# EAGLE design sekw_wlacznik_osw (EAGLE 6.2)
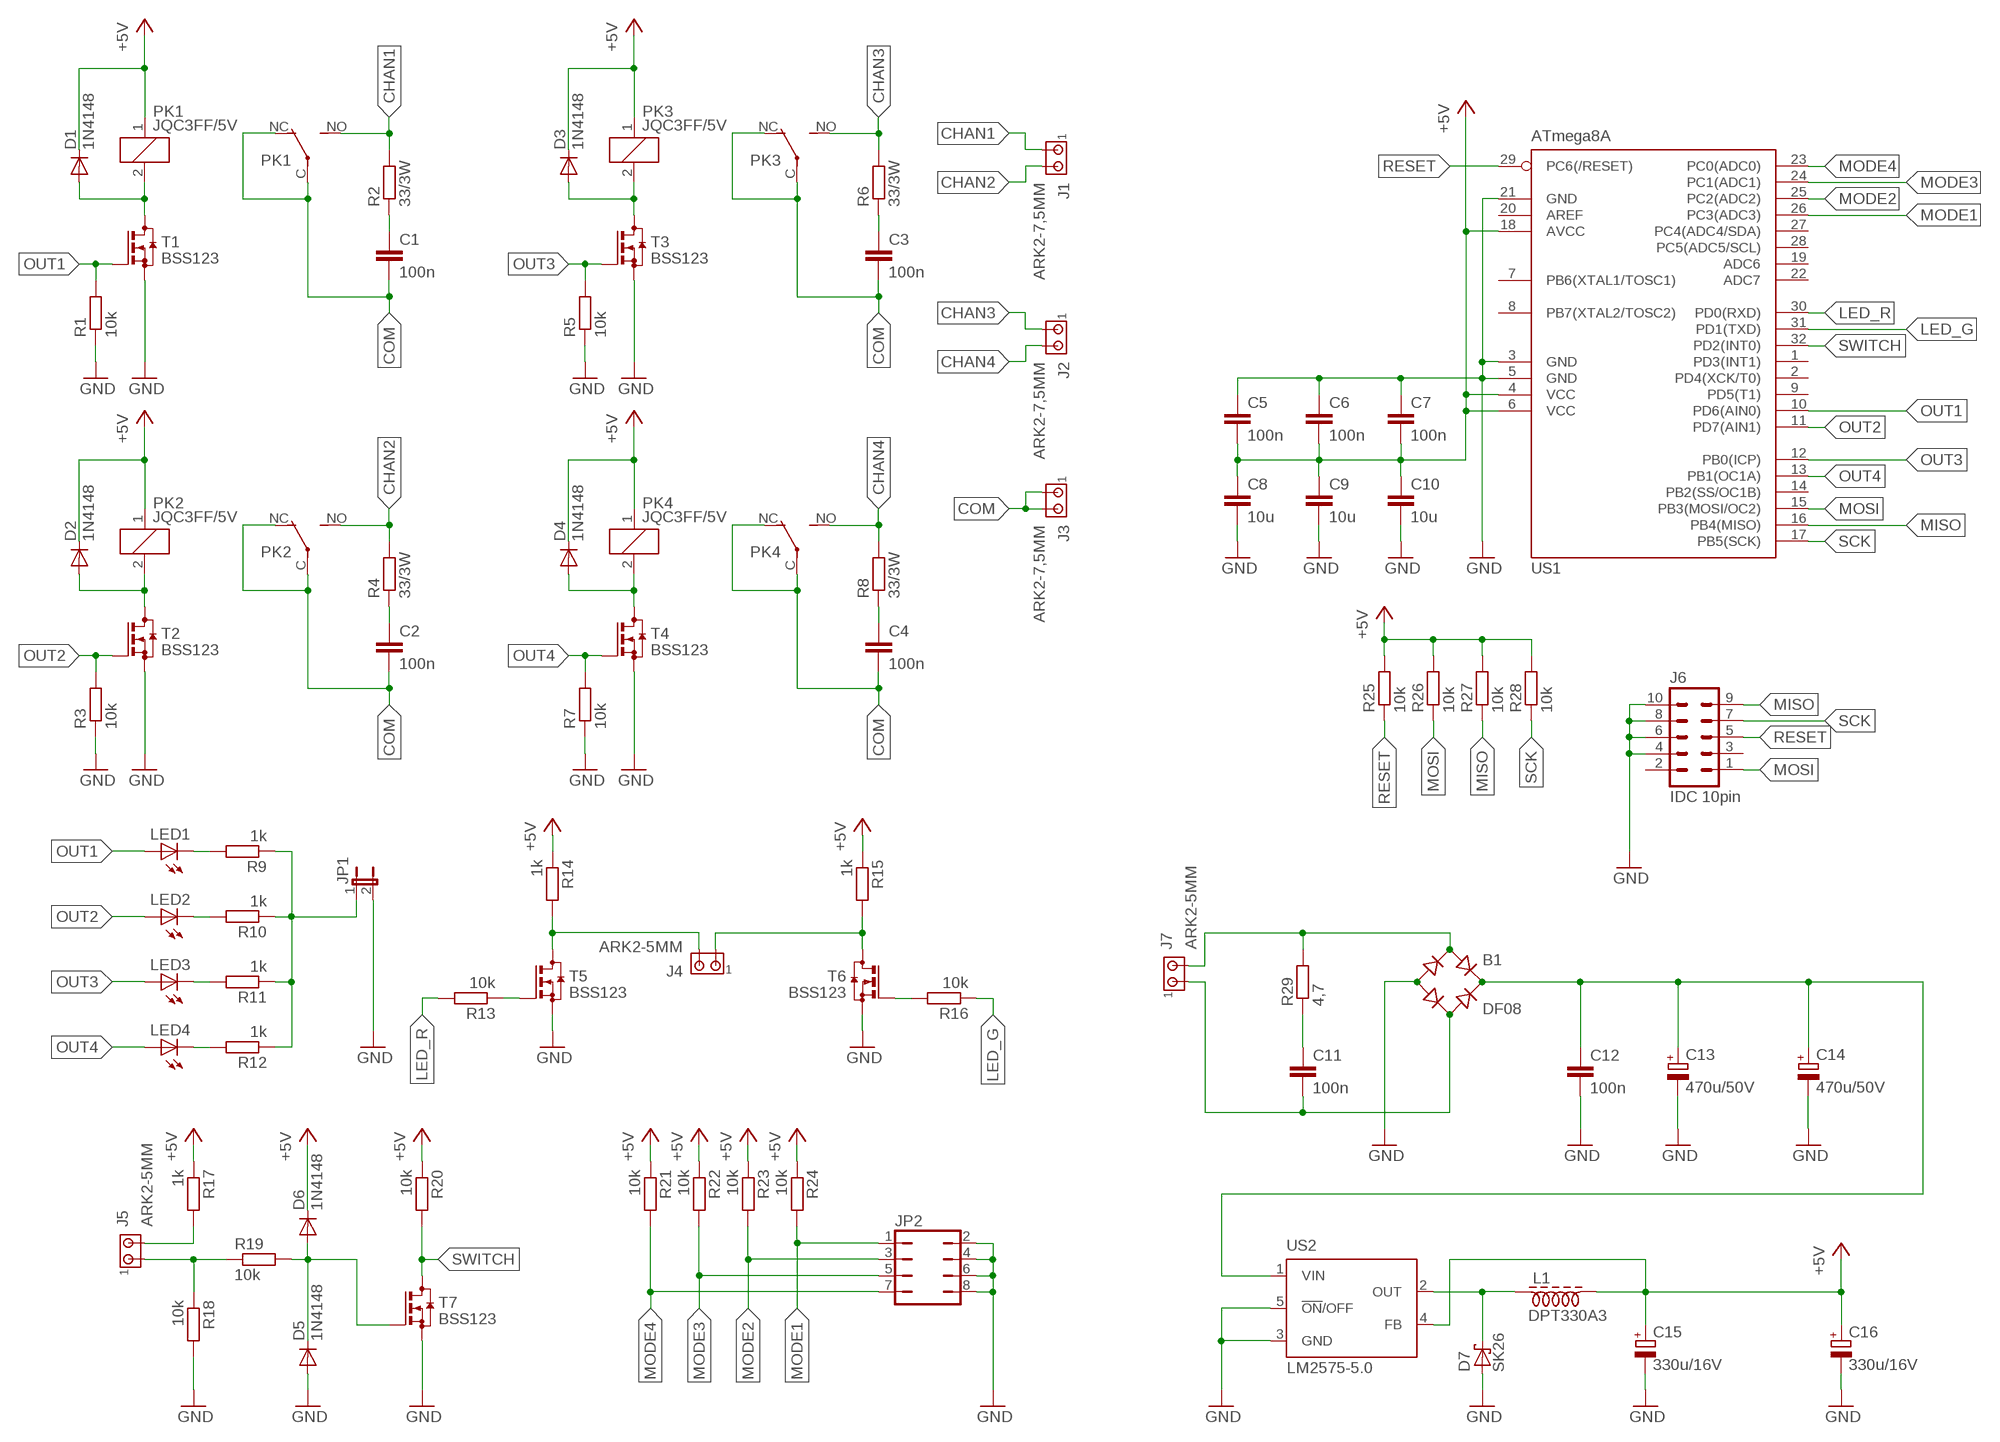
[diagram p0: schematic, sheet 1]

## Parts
B1  DF08  B-DIL  [B-DIL]
C1  100n  C-EU102_152-062X184  [C102_152-062X184]
C2  100n  C-EU102_152-062X184  [C102_152-062X184]
C3  100n  C-EU102_152-062X184  [C102_152-062X184]
C4  100n  C-EU102_152-062X184  [C102_152-062X184]
C5  100n  C-EUC0805  [C0805]
C6  100n  C-EUC0805  [C0805]
C7  100n  C-EUC0805  [C0805]
C8  10u  C-EUC0805  [C0805]
C9  10u  C-EUC0805  [C0805]
C10  10u  C-EUC0805  [C0805]
C11  100n  C-EUC0805  [C0805]
C12  100n  C-EUC0805  [C0805]
C13  470u/50V  CPOL-EUE5-10.5  [E5-10,5]
C14  470u/50V  CPOL-EUE5-10.5  [E5-10,5]
C15  330u/16V  CPOL-EUE3.5-8  [E3,5-8]
C16  330u/16V  CPOL-EUE3.5-8  [E3,5-8]
D1  1N4148  DIODE-MINIMELF  [MINIMELF]
D2  1N4148  DIODE-MINIMELF  [MINIMELF]
D3  1N4148  DIODE-MINIMELF  [MINIMELF]
D4  1N4148  DIODE-MINIMELF  [MINIMELF]
D5  1N4148  DIODE-MINIMELF  [MINIMELF]
D6  1N4148  DIODE-MINIMELF  [MINIMELF]
D7  SK26  SCHOTTKY-DIODESMD  [SMB]
J1  ARK2-7,5MM  [2PIN-7,5MM]
J2  ARK2-7,5MM  [2PIN-7,5MM]
J3  ARK2-7,5MM  [2PIN-7,5MM]
J4  ARK2-5MM  [2PIN-5MM]
J5  ARK2-5MM  [2PIN-5MM]
J6  IDC 10pin  ML10  [ML10]
J7  ARK2-5MM  [2PIN-5MM]
JP1  JP1E  [JP1]
JP2  JP4Q  [JP4Q]
L1  DPT330A3  DLAWIK-TOROID_16,5X9MM  [L_TOROID_16,5X9MM]
LED1  LEDCHIPLED_0805  [CHIPLED_0805]
LED2  LEDCHIPLED_0805  [CHIPLED_0805]
LED3  LEDCHIPLED_0805  [CHIPLED_0805]
LED4  LEDCHIPLED_0805  [CHIPLED_0805]
PK1  JQC3FF/5V  PK_POJED-JQC-3FG  [PK_POJED_JQC-3FG]
PK2  JQC3FF/5V  PK_POJED-JQC-3FG  [PK_POJED_JQC-3FG]
PK3  JQC3FF/5V  PK_POJED-JQC-3FG  [PK_POJED_JQC-3FG]
PK4  JQC3FF/5V  PK_POJED-JQC-3FG  [PK_POJED_JQC-3FG]
R1  10k  R-EU_R0805  [R0805]
R2  33/3W  R-EU_0613/5V  [P0613V]
R3  10k  R-EU_R0805  [R0805]
R4  33/3W  R-EU_0613/5V  [P0613V]
R5  10k  R-EU_R0805  [R0805]
R6  33/3W  R-EU_0613/5V  [P0613V]
R7  10k  R-EU_R0805  [R0805]
R8  33/3W  R-EU_0613/5V  [P0613V]
R9  1k  R-EU_R0805  [R0805]
R10  1k  R-EU_R0805  [R0805]
R11  1k  R-EU_R0805  [R0805]
R12  1k  R-EU_R0805  [R0805]
R13  10k  R-EU_R0805  [R0805]
R14  1k  R-EU_R0805  [R0805]
R15  1k  R-EU_R0805  [R0805]
R16  10k  R-EU_R0805  [R0805]
R17  1k  R-EU_R0805  [R0805]
R18  10k  R-EU_R0805  [R0805]
R19  10k  R-EU_R0805  [R0805]
R20  10k  R-EU_R0805  [R0805]
R21  10k  R-EU_R0805  [R0805]
R22  10k  R-EU_R0805  [R0805]
R23  10k  R-EU_R0805  [R0805]
R24  10k  R-EU_R0805  [R0805]
R25  10k  R-EU_R0805  [R0805]
R26  10k  R-EU_R0805  [R0805]
R27  10k  R-EU_R0805  [R0805]
R28  10k  R-EU_R0805  [R0805]
R29  4,7  R-EU_M1206  [M1206]
T1  BSS123  [SOT23]
T2  BSS123  [SOT23]
T3  BSS123  [SOT23]
T4  BSS123  [SOT23]
T5  BSS123  [SOT23]
T6  BSS123  [SOT23]
T7  BSS123  [SOT23]
US1  ATmega8A  MEGA8-AI  [TQFP32-08]
US2  LM2575-5.0  LM2596T  [T05D]

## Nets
+5V: C5.2 C6.2 C7.2 C8.1 C9.1 C10.1 C15.+ C16.+ D1.C D2.C D3.C D4.C D6.C L1.P$2 PK1.1 PK2.1 PK3.1 PK4.1 R14.1 R15.1 R17.1 R20.1 R21.1 R22.1 R23.1 R24.1 R25.2 R26.2 R27.2 R28.2 US1.4(VCC) US1.6(VCC) US1.18(AVCC) US2.4(FB)
CHAN1: J1.P1 PK1.NO R2.2
CHAN2: J1.P2 PK2.NO R4.2
CHAN3: J2.P1 PK3.NO R6.2
CHAN4: J2.P2 PK4.NO R8.2
COM: C1.2 C2.2 C3.2 C4.2 J3.P1 J3.P2 PK1.C(COM) PK1.NC PK2.C(COM) PK2.NC PK3.C(COM) PK3.NC PK4.C(COM) PK4.NC
GND: B1.- C5.1 C6.1 C7.1 C8.2 C9.2 C10.2 C12.2 C13.- C14.- C15.- C16.- D5.A D7.A J6.4 J6.6 J6.8 J6.10 JP1.2 JP2.2 JP2.4 JP2.6 JP2.8 R1.1 R3.1 R5.1 R7.1 R18.2 T1.2(S) T2.2(S) T3.2(S) T4.2(S) T5.2(S) T6.2(S) T7.2(S) US1.3(GND) US1.5(GND) US1.21(GND) US2.3(GND) US2.5(!ON!/OFF)
LED_G: R16.1 US1.31(PD1(TXD))
LED_R: R13.2 US1.30(PD0(RXD))
MISO: J6.9 R27.1 US1.16(PB4(MISO))
MODE1: JP2.1 R24.2 US1.26(PC3(ADC3))
MODE2: JP2.3 R23.2 US1.25(PC2(ADC2))
MODE3: JP2.5 R22.2 US1.24(PC1(ADC1))
MODE4: JP2.7 R21.2 US1.23(PC0(ADC0))
MOSI: J6.1 R26.1 US1.15(PB3(MOSI/OC2))
N$1: J4.P$1 R15.2 T6.3(D)
N$2: C1.1 R2.1
N$3: D1.A PK1.2 T1.3(D)
N$4: R16.2 T6.1(G)
N$5: C2.1 R4.1
N$6: D2.A PK2.2 T2.3(D)
N$7: C3.1 R6.1
N$8: D3.A PK3.2 T3.3(D)
N$9: C4.1 R8.1
N$10: D4.A PK4.2 T4.3(D)
N$11: J4.P$2 R14.2 T5.3(D)
N$12: R13.1 T5.1(G)
N$13: LED4.C R12.2
N$14: LED3.C R11.2
N$15: LED2.C R10.2
N$16: LED1.C R9.2
N$17: JP1.1 R9.1 R10.1 R11.1 R12.1
N$18: J5.P$2 R17.2
N$19: J5.P$1 R18.1 R19.1
N$20: D5.C D6.A R19.2 T7.1(G)
N$21: B1.AC2 C11.2 J7.P$1
N$22: B1.AC1 J7.P$2 R29.2
N$23: C11.1 R29.1
N$24: B1.+ C12.1 C13.+ C14.+ US2.1(VIN)
N$25: D7.C L1.P$1 US2.2(OUT)
OUT1: LED1.A R1.2 T1.1(G) US1.10(PD6(AIN0))
OUT2: LED2.A R3.2 T2.1(G) US1.11(PD7(AIN1))
OUT3: LED3.A R5.2 T3.1(G) US1.12(PB0(ICP))
OUT4: LED4.A R7.2 T4.1(G) US1.13(PB1(OC1A))
RESET: J6.5 R25.1 US1.29(PC6(/RESET))
SCK: J6.7 R28.1 US1.17(PB5(SCK))
SWITCH: R20.2 T7.3(D) US1.32(PD2(INT0))
Unconnected: J6.2 J6.3 US1.1(PD3(INT1)) US1.2(PD4(XCK/T0)) US1.7(PB6(XTAL1/TOSC1)) US1.8(PB7(XTAL2/TOSC2)) US1.9(PD5(T1)) US1.14(PB2(SS/OC1B)) US1.19(ADC6) US1.20(AREF) US1.22(ADC7) US1.27(PC4(ADC4/SDA)) US1.28(PC5(ADC5/SCL))

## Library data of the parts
B1 = rectifier:B-DIL: RECTIFIER
C1-C4 = resistor:C-EU: CAPACITOR, European symbol
C5-C12 = rcl:C-EU: CAPACITOR, European symbol
C13-C16 = rcl:CPOL-EU: POLARIZED CAPACITOR, European symbol
D1-D6 = diode:DIODE-: DIODE
D7 = diode:SCHOTTKY-DIODE: Schottky Diode
J1-J5 J7 = zlacza_futrzak:ARK2: ARK 2
J6 = con-harting-ml:ML10: HARTING; OC_FARNELL: unknown; OC_NEWARK: unknown
JP1 = jumper:JP1E: JUMPER
JP2 = jumper:JP4Q: JUMPER
L1 = inne_futrzak:DLAWIK
LED1-LED4 = led:LED: LED
PK1-PK4 = inne_futrzak:PK_POJED
R1 R3 R5 R7 R9-R29 = rcl:R-EU_: RESISTOR, European symbol
R2 R4 R6 R8 = resistor:R-EU_: RESISTOR, European symbol
T1-T7 = transistor-small-signal:BSS123: N-CHANNEL MOS FET
US1 = atmel:MEGA8: MICROCONTROLLER 8 Kbytes FLASH, 1 kbytes SRAM, 512 bytes EEPROM, USART, 6-channel 10 bit ADC, 2-channel 8 bit ADC Pin compatible with Atmega48, ATMega88, ATMega168 Source: avr.lbr; MPN: ATMEGA8-16AU; OC_FARNELL: 9171371; OC_NEWARK: 73M8863
US2 = national-semiconductor:LM2596: SIMPLE SWITCHER® Power Converter 150 kHz 3A Step-Down Voltage Regulator Source: http://www.national.com/ds/LM/LM2596.pdf; MPN: LM2596T-ADJ/LF02; OC_FARNELL: 9494162; OC_NEWARK: 65K5910

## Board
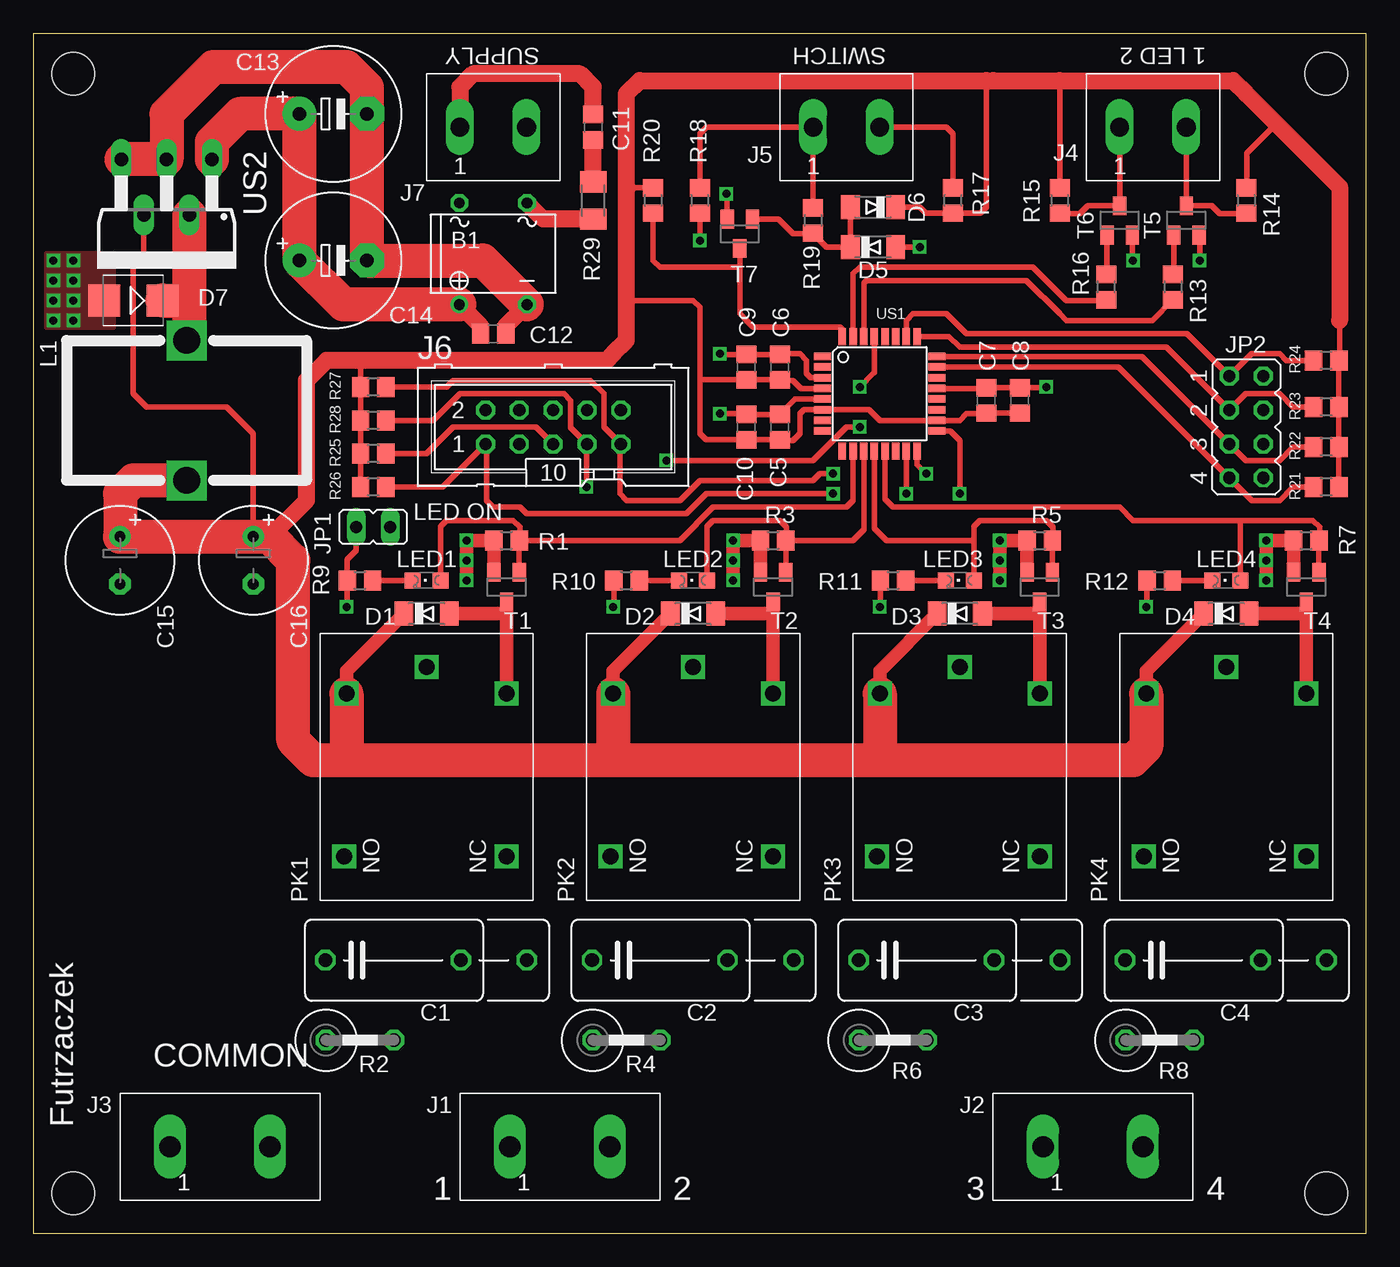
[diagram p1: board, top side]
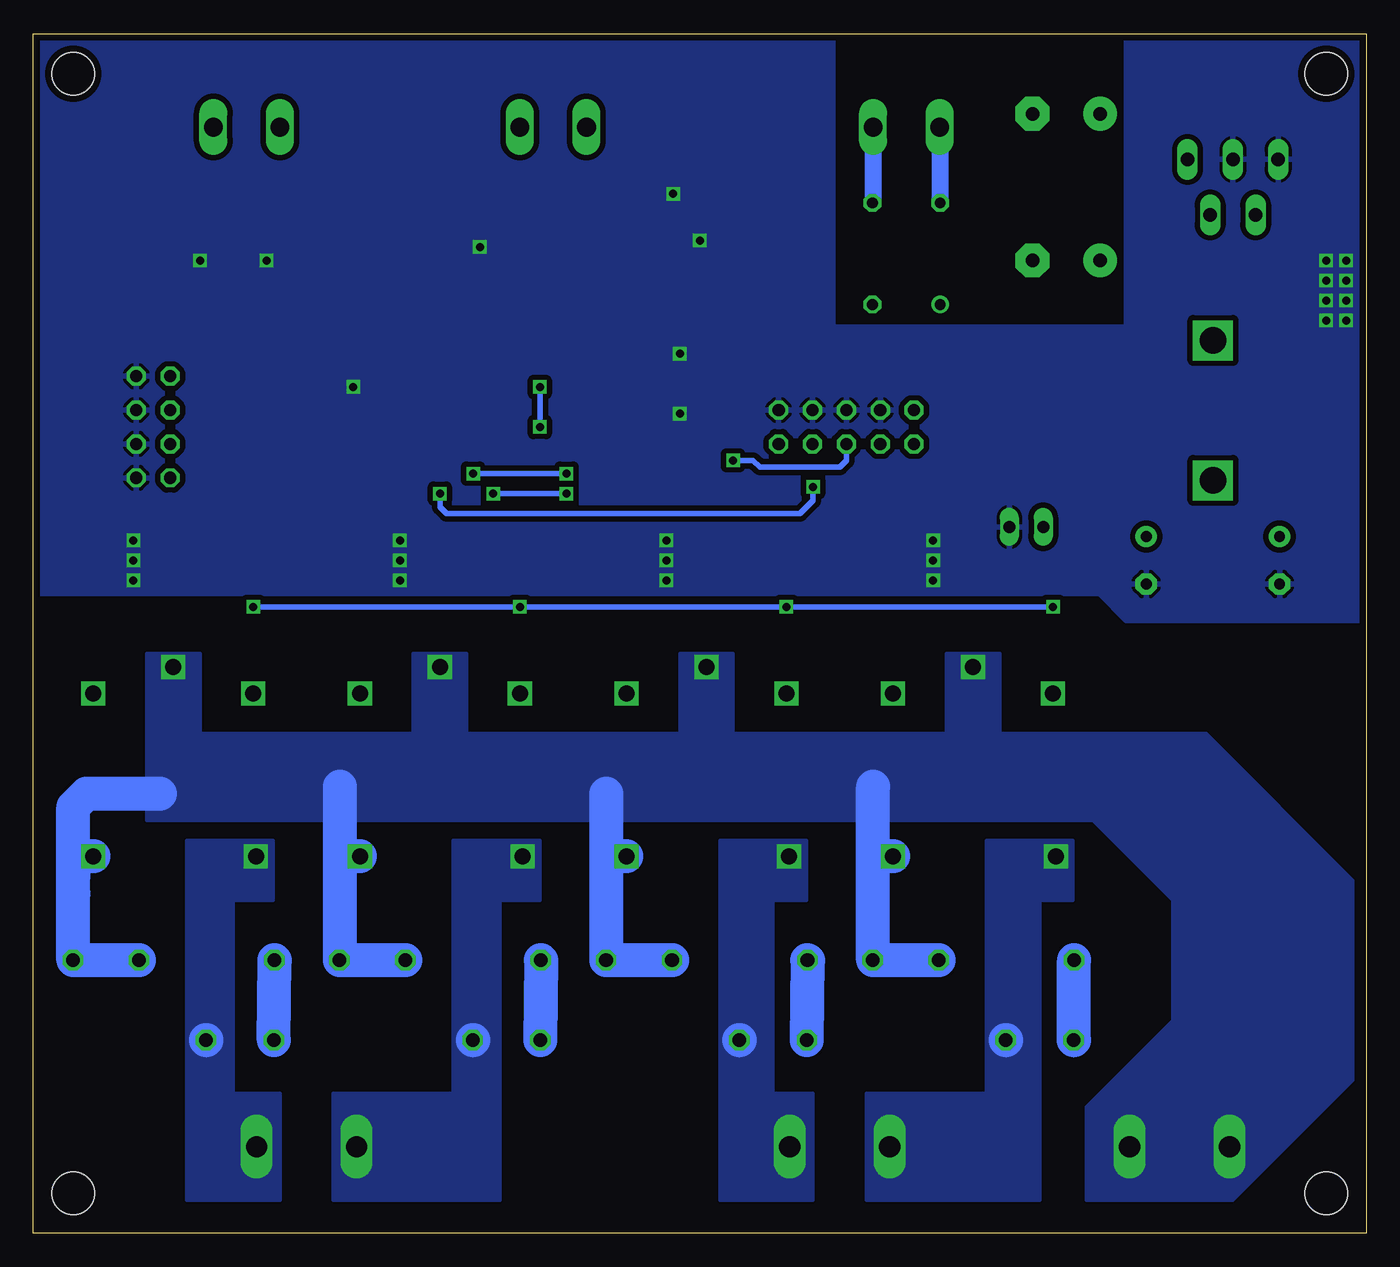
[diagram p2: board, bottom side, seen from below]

Size 100 x 90 mm. Coordinates in mm from the lower left corner, seen from the top.
Outline: 0,0 100,0 100,90 0,90 0,0
Copper layers (1*16): Top 0.035mm / dielectric 1.5mm / Bottom 0.035mm
Design rules: minimum track width 10mil, minimum drill 23mil, track to track 8mil, track to pad 8mil, pad to pad 8mil, via to via 8mil, smd to smd 8mil, copper to edge 20mil, drill to drill 8mil, minimum pad ring 10mil, minimum via ring 8mil, stop-mask expansion 4mil, vias tented up to drill 0mil, thermal gap 10mil
Holes 3.2 mm at 3,3 97,3 3,87 97,87

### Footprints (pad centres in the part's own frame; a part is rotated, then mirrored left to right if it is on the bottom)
B-DIL = drill 0.813: + -2.54,-3.81 | drill 0.813 octagon: - 2.54,-3.81; AC1 2.54,3.81; AC2 -2.54,3.81
C102_152-062X184 = drill 1.016 octagon: 1 -5.08,0; 2 5.08,0; 3 10.033,0
C0805 = smd 1.3 x 1.5: 1 -0.95,0; 2 0.95,0
E5-10,5 = drill 1.016 pad 2.54: + -2.54,0 | drill 1.016 pad 2.54 octagon: - 2.54,0
E3,5-8 = drill 0.813 pad 1.6: + -1.778,0 | drill 0.813 pad 1.6 octagon: - 1.778,0
MINIMELF = smd 1.4 x 1.8: A 1.7,0; C -1.7,0
SMB = smd 2.4 x 2.4: A 2.2,0; C -2.2,0
2PIN-7,5MM = drill 1.6 long: P1 -3.75,0; P2 3.75,0
2PIN-5MM = drill 1.4 long: P$1 -2.5,0; P$2 2.5,0
ML10 = drill 0.914 octagon: 1 -5.08,-1.27; 2 -5.08,1.27; 3 -2.54,-1.27; 4 -2.54,1.27; 5 0,-1.27; 6 0,1.27; 7 2.54,-1.27; 8 2.54,1.27; 9 5.08,-1.27; 10 5.08,1.27
JP1 = drill 0.914 long: 1 0,-1.27; 2 0,1.27
JP4Q = drill 0.914 octagon: 1 -3.81,-1.27; 2 -3.81,1.27; 3 -1.27,-1.27; 4 -1.27,1.27; 5 1.27,-1.27; 6 1.27,1.27; 7 3.81,-1.27; 8 3.81,1.27
L_TOROID_16,5X9MM = drill 2 square: P$1 -5,0; P$2 5.5,0
CHIPLED_0805 = smd 1.2 x 1.2: A 0,-1.05; C 0,1.05
PK_POJED_JQC-3FG = drill 1.2 square: 1 5.5,6; 2 5.5,-6; C 7.5,0; NC -6.7,-6; NO -6.7,6.2
R0805 = smd 1.3 x 1.5: 1 -0.95,0; 2 0.95,0
P0613V = drill 1.016 octagon: 1 -2.54,0; 2 2.54,0
M1206 = smd 1.6 x 2: 1 -1.4,0; 2 1.4,0
SOT23 = smd 1 x 1.4: 1 -0.95,-1.1; 2 0.95,-1.1; 3 0,1.1
TQFP32-08 = smd 1.27 x 0.559: 1 -4.293,2.8; 2 -4.293,2; 3 -4.293,1.2; 4 -4.293,0.4; 5 -4.293,-0.4; 6 -4.293,-1.2; 7 -4.293,-2; 8 -4.293,-2.8; 17 4.293,-2.8; 18 4.293,-2; 19 4.293,-1.2; 20 4.293,-0.4; 21 4.293,0.4; 22 4.293,1.2; 23 4.293,2; 24 4.293,2.8 | smd 0.559 x 1.27: 9 -2.8,-4.293; 10 -2,-4.293; 11 -1.2,-4.293; 12 -0.4,-4.293; 13 0.4,-4.293; 14 1.2,-4.293; 15 2,-4.293; 16 2.8,-4.293; 25 2.8,4.293; 26 2,4.293; 27 1.2,4.293; 28 0.4,4.293; 29 -0.4,4.293; 30 -1.2,4.293; 31 -2,4.293; 32 -2.8,4.293
T05D = drill 1.016 long: 1 -3.404,-5.08; 2 -1.702,-0.914; 3 0,-5.08; 4 1.702,-0.914; 5 3.404,-5.08

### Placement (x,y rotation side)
B1  34.5,73.5 0 top
C1  27,20.5 0 top
C2  47,20.5 0 top
C3  67,20.5 0 top
C4  87,20.5 0 top
C5  56,60.5 270 top
C6  56,65 270 top
C7  71.5,62.5 270 top
C8  74,62.5 90 top
C9  53.5,65 90 top
C10  53.5,60.5 90 top
C11  42,83 90 top
C12  34.5,67.5 0 top
C13  22.5,84 0 top
C14  22.5,73 0 top
C15  6.5,50.5 270 top
C16  16.5,50.5 270 top
D1  29.5,46.5 0 top
D2  49.5,46.5 0 top
D3  69.5,46.5 0 top
D4  89.5,46.5 0 top
D5  63,74 0 top
D6  63,77 180 top
D7  7.5,70 180 top
J1  39.5,6.5 0 top
J2  79.5,6.5 0 top
J3  14,6.5 0 top
J4  84,83 0 top
J5  61,83 0 top
J6  39,60.5 0 top
J7  34.5,83 0 top
JP1  25.5,53 270 top
JP2  91,60.5 270 top
L1  11.5,62 270 top
LED1  29.5,49 90 top
LED2  49.5,49 90 top
LED3  69.5,49 90 top
LED4  89.5,49 90 top
PK1  29.5,35 90 top
PK2  49.5,35 90 top
PK3  69.5,35 90 top
PK4  89.5,35 90 top
R1  35.5,52 0 top
R2  24.5,14.5 0 top
R3  55.5,52 0 top
R4  44.5,14.5 0 top
R5  75.5,52 0 top
R6  64.5,14.5 0 top
R7  95.5,52 0 top
R8  84.5,14.5 0 top
R9  24.5,49 0 top
R10  44.5,49 0 top
R11  64.5,49 0 top
R12  84.5,49 0 top
R13  85.5,71 270 top
R14  91,77.5 270 top
R15  77,77.5 270 top
R16  80.5,71 90 top
R17  69,77.5 90 top
R18  50,77.5 270 top
R19  58.5,76 270 top
R20  46.5,77.5 270 top
R21  97,56 180 top
R22  97,59 180 top
R23  97,62 180 top
R24  97,65.5 180 top
R25  25.5,58.5 180 top
R26  25.5,56 180 top
R27  25.5,63.5 180 top
R28  25.5,61 180 top
R29  42,77.5 270 top
T1  35.5,48.5 180 top
T2  55.5,48.5 180 top
T3  75.5,48.5 180 top
T4  95.5,48.5 180 top
T5  86.5,76 0 top
T6  81.5,76 0 top
T7  53,75 180 top
US1  63.5,63 0 top
US2  10,75.5 180 top

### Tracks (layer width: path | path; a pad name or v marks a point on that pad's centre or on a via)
+5V
  Top 0.406: US2.4 8.3,73.3 7.5,72.5 7.5,63 8.5,62 14.5,62 16.5,60 C16.+ | R15.1 77,86.5 72,86.5 | D6.C 66.5,77 66.95,76.55 R17.1 71.05,76.55 71.5,77 71.5,86.5 | R20.1 44.55,78.45 44.5,78.5 | R21.1 R22.1 R23.1 R24.1 98,65.55 98,68.5 | R14.1 91.05,78.5 91.05,81.05 93.25,83.25 | US1.4 57.6,63.4 57,64 56.05,64 C6.2 C9.1 50.55,64.05 50.05,64.05 50,64 | C8.1 C7.2 71.45,61.5 70,61.5 69.5,61 US1.18 63.5,61 62.7,61.8 US1.6 57.8,61.8 57.5,61.5 57.5,60 57,59.5 56.05,59.5 C5.2 C10.1 50.45,59.55 50,60 50,63.5 50,64 | 50,64 50,69.5 49.5,70 45,70 44.5,69.5 | R26.2 R25.2 R28.2 R27.2 24.55,64.95 24,65.5
  Top 1.016: PK4.1 83.5,42.2 D4.C | PK3.1 63.5,42.2 D3.C | D2.C 43.5,42.2 PK2.1 | D1.C 23.5,42.2 PK1.1
  Top 1.27: 17.72,52.28 17.78,52.28 20.5,55 20.5,64 22,65.5 24,65.5 43,65.5 43.5,66 44.5,67 44.5,69.5 44.5,78.4 44.55,78.45 | 44.5,78.5 44.5,85.5 45.5,86.5 71.5,86.5 72,86.5 77,86.5 90,86.5 91,85.5 93.25,83.25 98,78.5 98,68.5
  Top 2.54: PK4.1 83.5,36.5 82.5,35.5 63.5,35.5 | 63.5,35.5 43.5,35.5 | 43.5,35.5 23.5,35.5 | PK3.1 63.5,35.5 | PK2.1 43.5,35.5 | PK1.1 23.5,35.5 | 23.5,35.5 21,35.5 19.5,37 19.5,50.5 17.72,52.28 C16.+ C15.+ 6.5,55.5 7.5,56.5 L1.P$2
CHAN1
  Bottom 2.54: R2.2 27,14.5
  pour Bottom (no thermals): 22,29.5 22,25 24.5,25 24.5,2.5 37.5,2.5 37.5,10.5 28.5,10.5 28.5,29.5
CHAN2
  Bottom 2.54: R4.2 47,14.5
  pour Bottom (no thermals): 42,29.5 42,25 44.5,25 44.5,10.5 41.5,10.5 41.5,2.5 48.5,2.5 48.5,29.5
CHAN3
  Bottom 2.54: R6.2 67,14.5
  pour Bottom (no thermals): 62,29.5 62,25 65,25 65,2.5 77.5,2.5 77.5,10.5 68.5,10.5 68.5,29.5
CHAN4
  Bottom 2.54: R8.2 87,14.5
  pour Bottom (no thermals): 82,29.5 82,25 85,25 85,10.5 81.5,10.5 81.5,2.5 88.5,2.5 88.5,29.5
COM
  Bottom 2.54: C1.2 37,20.5 37,28.5 | 37,28.5 37,33.5 | PK1.NC 37,28.3 37,28.5 | C2.2 57,20.5 57,28.5 | 57,28.5 57,33 | PK2.NC 57,28.3 57,28.5 | C3.2 77,20.5 77,28.5 | 77,28.5 77,33.5 | PK3.NC 77,28.3 77,28.5 | C4.2 97,20.5 97,25.5 97,26.8 97,28.5 | 97,28.5 97,32 96,33 90.5,33 | PK4.NC 96.8,28.3 97,28.5
  pour Bottom (no thermals): 21,2.5 10,2.5 1,11.5 1,26.5 12,37.5 27.5,37.5 27.5,43.5 31.5,43.5 31.5,37.5 47.5,37.5 47.5,43.5 51.5,43.5 51.5,37.5 67.5,37.5 67.5,43.5 71.5,43.5 71.5,37.5 87.5,37.5 87.5,43.5 91.5,43.5 91.5,31 20.5,31 14.5,25 14.5,16 21,9.5
GND  (via drill 0.6)
  Top 0.406: T6.2 82.45,73.05 v82.5,73 | v87.5,73 87.5,74.85 T5.2 | R18.2 v50,74.5 | D5.A v66.5,74 | T7.2 52.05,77.95 v52,78 | v51.5,66 51.55,65.95 C9.2 C6.1 56.05,66 57.5,66 58,65.5 58,64.5 58.3,64.2 US1.3 | v51.5,61.5 53.45,61.5 C10.2 C5.1 57.15,62.6 US1.5 | v76,63.5 75.95,63.45 C8.2 C7.1 71.45,63.4 US1.21
  Top 1.016: v32.5,49 v32.5,50.5 v32.5,52 R1.1 T1.2 | v52.5,49 v52.5,50.5 v52.5,52 R3.1 T2.2 | v72.5,49 v72.5,50.5 v72.5,52 R5.1 T3.2 | v92.5,49 v92.5,50.5 v92.5,52 R7.1 T4.2
  Top 1.27: C12.2 35.45,68.1 B1.-
  Top 2.54: B1.- 33.73,73 C14.- C13.- 25.04,85.96 23.5,87.5 13.5,87.5 10,84 US2.3 US2.5
  other vias: 3,73 3,71.5 3,70 3,68.5 1.5,68.5 1.5,70 1.5,71.5 1.5,73
  pour Top (no thermals): 1,73.5 6,73.5 6,68 1,68
  pour Bottom (isolate 0.406): 0,90 18,90 18,68 40,68 40,90 100,90 100,48 20,48 18,46 0,46
LED_G
  Top 0.406: US1.31 61.5,72 62,72.5 75,72.5 77.5,70 80.45,70 R16.1
LED_R
  Top 0.406: US1.30 62.3,71.3 62.5,71.5 74.5,71.5 77,69 77.5,68.5 83.95,68.5 R13.2
MISO  (via drill 0.6)
  Top 0.406: R27.1 31,63.5 31.5,64 41.8,64 42.8,63 42.8,60.51 J6.9 44,59.15 44,55.5 44.5,55 48.5,55 50,56.5 58.5,56.5 59,57 v60,57 | US1.16 66.3,57.7 v67,57
  Bottom 0.406: v67,57 v60,57
MODE1
  Top 0.406: R24.2 94,65.5 93.5,66 91.42,66 JP2.1 86.54,67.5 70,67.5 68.5,69 66,69 65.5,68.5 US1.26
MODE2
  Top 0.406: R23.2 94.5,62 93.5,63 90.96,63 JP2.3 85,66.5 69.5,66.5 68.71,67.29 US1.25
MODE3
  Top 0.406: R22.2 94.5,59 93.5,58 90.96,58 JP2.5 83.16,65.8 US1.24
MODE4
  Top 0.406: R21.2 94.5,56 93.5,55 91.42,55 JP2.7 81.42,65 US1.23
MOSI  (via drill 0.6)
  Top 0.406: R26.1 30.69,56 J6.1 34,59.15 34,55 34.5,54.5 36.5,54.5 37,54 49,54 50.5,55.5 v60,55.5 | US1.15 v65.5,55.5
  Bottom 0.406: v65.5,55.5 v60,55.5
N$1
  Top 0.406: J4.P$1 T6.3 79.1,77.1 78.5,76.5 77.05,76.5 R15.2
N$2
  Bottom 2.54: R2.1 21.92,14.5 C1.1
N$3
  Top 1.016: PK1.2 35.5,46.5 | 35.5,46.5 T1.3 | D1.A 35.5,46.5
N$4
  Top 0.406: T6.1 80.55,72 R16.2
N$5
  Bottom 2.54: R4.1 41.88,20.46 C2.1
N$6
  Top 1.016: PK2.2 55.5,46.5 | 55.5,46.5 T2.3 | D2.A 55.5,46.5
N$7
  Bottom 2.54: R6.1 61.88,20.46 C3.1
N$8
  Top 1.016: PK3.2 75.5,46.5 | 75.5,46.5 T3.3 | D3.A 75.5,46.5
N$9
  Bottom 2.54: R8.1 81.88,20.46 C4.1
N$10
  Top 1.016: PK4.2 95.5,46.5 | 95.5,46.5 T4.3 | D4.A 95.5,46.5
N$11
  Top 0.406: J4.P$2 T5.3 88.4,77.1 89,76.5 90.95,76.5 R14.2
N$12
  Top 0.406: T5.1 85.55,72 R13.1
N$13
  Top 0.406: R12.2 LED4.C
N$14
  Top 0.406: R11.2 LED3.C
N$15
  Top 0.406: R10.2 LED2.C
N$16
  Top 0.406: R9.2 LED1.C
N$17  (via drill 0.6)
  Top 0.406: v23.5,47 23.55,47.05 R9.1 23.55,50.55 24,51 24.23,51.23 JP1.1 | R10.1 43.55,47.05 v43.5,47 | R11.1 63.55,47.05 v63.5,47 | R12.1 83.55,47.05 v83.5,47
  Bottom 0.406: v83.5,47 v63.5,47 v43.5,47 v23.5,47
N$18
  Top 0.406: J5.P$2 68.5,83 69,82.5 R17.2
N$19
  Top 0.406: R19.1 J5.P$1 50.5,83 50,82.5 R18.1
N$20
  Top 0.406: D6.A D5.C 59.5,74 58.5,75 R19.2 58.45,75 57,75 55.9,76.1 T7.1
N$21
  Top 1.27: C11.2 42,86 41,87 33,87 32,86 J7.P$1
  Bottom 1.27: J7.P$1 32,77.35 B1.AC2
N$22
  Top 1.27: R29.2 38.25,76.1 B1.AC1
  Bottom 1.27: J7.P$2 37,77.35 B1.AC1
N$23
  Top 1.27: R29.1 C11.1
N$24
  Top 1.27: C12.1 33.55,68.1 B1.+
  Top 2.54: B1.+ 23.27,69.69 C14.+ C13.+ 15.5,84 13.4,81.9 US2.1
N$25
  Top 2.54: US2.2 11.7,70 | 11.7,70 11.7,67.2 L1.P$1 | D7.C 11.7,70
OUT1
  Top 0.406: T1.1 R1.2 | LED1.A 30.55,53.05 31,53.5 36,53.5 36.5,53 36.5,52.05 R1.2 | US1.10 61.5,55 61,54.5 51,54.5 48.5,52 R1.2
OUT2
  Top 0.406: T2.1 R3.2 | LED2.A 50.55,53.05 51,53.5 56,53.5 56.5,53 56.5,52.05 R3.2 | US1.11 62.3,52.8 61.5,52 R3.2
OUT3
  Top 0.406: T3.1 R5.2 76.5,52.05 76.5,53 76,53.5 71,53.5 70.55,53.05 70.55,52 | LED3.A 70.55,52 | US1.12 63.1,52.9 64,52 70.55,52
OUT4
  Top 0.406: T4.1 R7.2 96.5,52.05 96.5,53 96,53.5 91,53.5 90.5,53.5 | LED4.A 90.55,52 90.55,53.05 90.55,53.45 90.5,53.5 | US1.13 63.9,55.1 64.5,54.5 81.5,54.5 82.5,53.5 90.5,53.5
RESET  (via drill 0.6)
  Top 0.406: US1.29 63.1,64.6 63,64.5 v62,63.5 | R25.1 29.5,58.5 31.5,60.5 37.73,60.5 J6.5 | v62,60.5 61,60.5 58.5,58 49,58 v47.5,58
  Bottom 0.406: v62,63.5 v62,60.5 | v47.5,58 46,58 45.5,57.5 39.5,57.5 39,58 J6.5
SCK  (via drill 0.6)
  Top 0.406: R28.1 30,61 32,63 39.8,63 40.3,62.5 40.3,60.47 J6.7 41.5,59.19 v41.5,56 | US1.17 68.8,60.2 69.5,59.5 v69.5,55.5
  Bottom 0.406: v69.5,55.5 69.5,54.5 69,54 42.5,54 41.5,55 v41.5,56
SWITCH
  Top 0.406: R20.2 46.5,73 47,72.5 52.5,72.5 53,72.5 | US1.32 60.7,67.8 60.5,68 54,68 53.5,68.5 53,69 53,72.5 | 53,72.5 T7.3

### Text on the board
tPlace: SUPPLY | SWITCH | 1 LED 2 | LED ON | COMMON | Futrzaczek | 1 | 2 | 3 | 4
